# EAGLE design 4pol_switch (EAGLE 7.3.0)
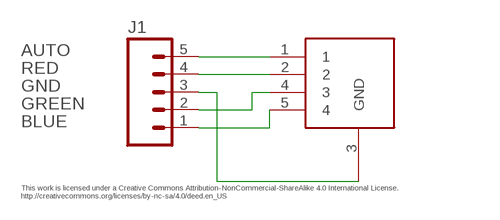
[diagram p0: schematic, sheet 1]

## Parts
J1  M05PTH  [1X05]
U$1  SK-14D07-VG  4POL-SLIDE-SWITCH  [4POLE_SLIDE_SWITCH]

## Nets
AUTO: J1.5 U$1.1
BLUE: J1.1 U$1.5
GND: J1.3 U$1.3(GND)
GREEN: J1.2 U$1.4
RED: J1.4 U$1.2

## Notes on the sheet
- AUTO
- RED
- GND
- GREEN
- BLUE
- This work is licensed under a Creative Commons Attribution-NonCommercial-ShareAlike 4.0 International License.
  http://creativecommons.org/licenses/by-nc-sa/4.0/deed.en_US

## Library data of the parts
J1 = SparkFun-Connectors:M05: Header 5 Standard 5-pin 0.1" header. Use with straight break away headers (SKU : PRT-00116), right angle break away headers (PRT-00553), swiss pins (PRT-00743), machine pins (PRT-00117), and female headers (PRT-00115). Molex polarized connector foot print use with SKU : PRT-08230 with associated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
U$1 = 4pole_slide_switch:4POL-SLIDE-SWITCH

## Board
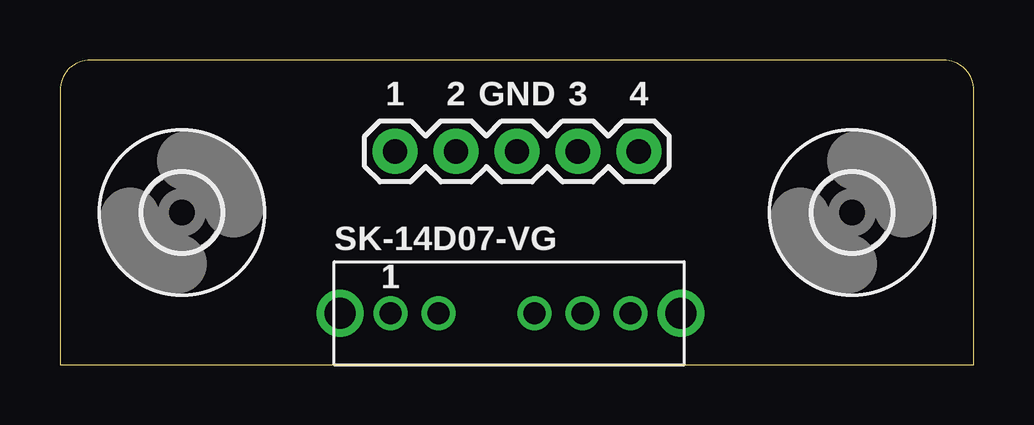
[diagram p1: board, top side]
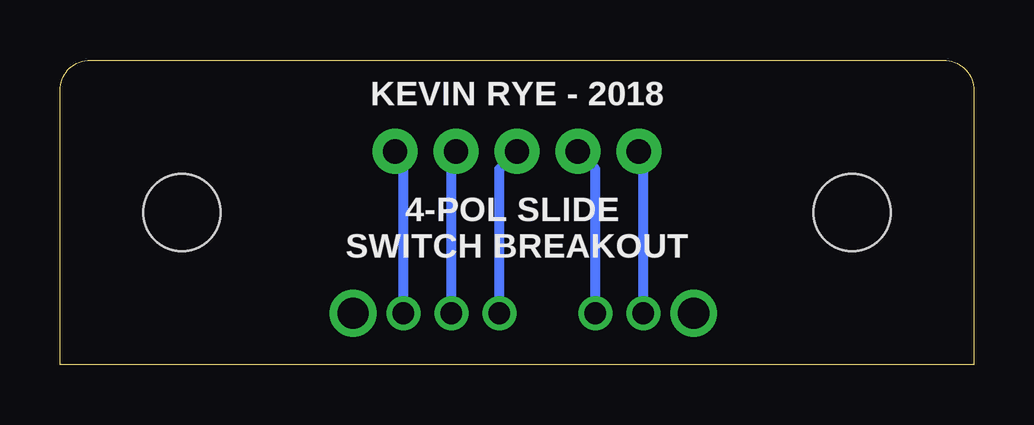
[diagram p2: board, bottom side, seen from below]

Size 38.1 x 12.7 mm. Coordinates in mm from the lower left corner, seen from the top.
Outline: 0,0 38.1,0 38.1,11.43 arc90 36.83,12.7 1.27,12.7 arc90 0,11.43 0,0
Copper layers (1*16): Top 0.035mm / dielectric 1.5mm / Bottom 0.035mm
Design rules "default": minimum track width 10mil, minimum drill 24mil, track to track 8mil, track to pad 8mil, pad to pad 8mil, via to via 8mil, smd to smd 8mil, copper to edge 40mil, drill to drill 8mil, minimum pad ring 10mil, minimum via ring 8mil, stop-mask expansion 4mil, vias tented up to drill 0mil, thermal gap 10mil

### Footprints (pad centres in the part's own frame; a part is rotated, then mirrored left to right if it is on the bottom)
1X05 = drill 1.016 pad 1.88: 1 0,0; 2 2.54,0; 3 5.08,0; 4 7.62,0; 5 10.16,0
4POLE_SLIDE_SWITCH = drill 0.9: 1 2.35,2.15; 2 4.35,2.15; 3 8.35,2.15; 4 10.35,2.15; 5 12.35,2.15 | drill 1.3: P$1 0.25,2.15; P$2 14.45,2.15
3,2 = hole 3.2: 0,0

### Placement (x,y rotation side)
J1  24.13,8.89 180 top
U$1  11.43,0 0 top
U$2  [3,2]  5.08,6.35 0 top
U$3  [3,2]  33.02,6.35 0 top

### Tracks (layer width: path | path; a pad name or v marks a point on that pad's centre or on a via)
AUTO
  Bottom 0.406: U$1.1 13.78,8.7 J1.5
BLUE
  Bottom 0.406: U$1.5 23.78,8.54 J1.1
GND
  Bottom 0.406: U$1.3 19.78,8.16 J1.3
GREEN
  Bottom 0.406: U$1.4 21.78,8.7 J1.2
RED
  Bottom 0.406: U$1.2 15.78,8.16 J1.4

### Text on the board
Unrouted: This work is licensed under a Creative Commons Attribution-NonCommercial-ShareAlike 4.0 International License. / http://creativecommons.org/licenses/by-nc-sa/4.0/deed.en_US
tPlace: SK-14D07-VG
tNames: 1 | 2 | GND | 3 | 4
bNames: KEVIN RYE - 2018 | 4-POL SLIDE / SWITCH BREAKOUT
